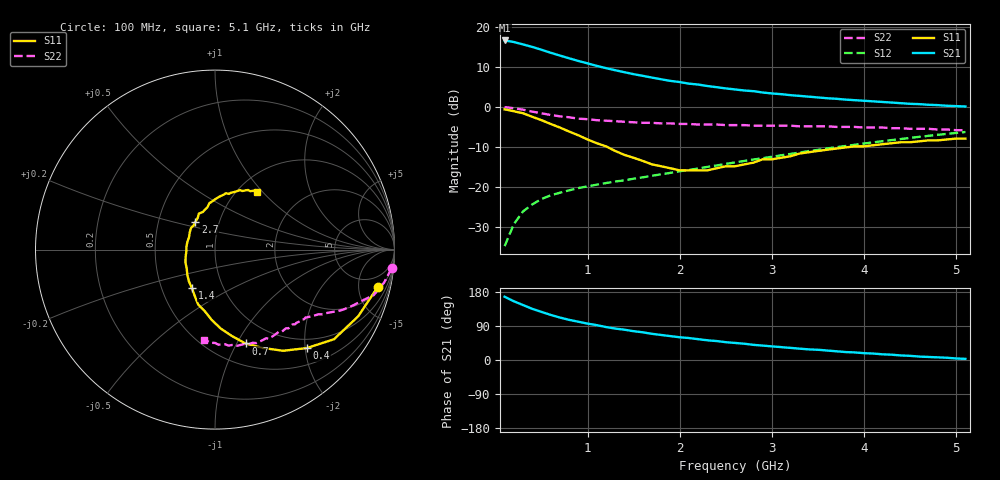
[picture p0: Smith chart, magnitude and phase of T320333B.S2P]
!AT-32033
!S and NOISE PARAMETERS at Vce=2.7V  Ic=2mA.  LAST UPDATED 01-05-95
# ghz s ma r 50
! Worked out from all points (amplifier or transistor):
!   51 points, 100 MHz to 5.1 GHz, reference 50 ohm
!   highest |S21| = 16.6 dB at 100 MHz (marker M1)
!   |S21| within 3 dB of that: start of sweep to 589.7 MHz
!   unconditionally stable (mu >= 1): 1.71 GHz to 2.774 GHz
!   at 900 MHz: K = 0.72, MSG = 15.9 dB, |S12| = -20.4 dB
!   at 2.6 GHz: K = 1.02, MAG = 8.3 dB, |S12| = -13.9 dB
!   at 5.1 GHz: K = 0.86, MSG = 3.2 dB, |S12| = -6.3 dB
!   lowest NFmin = 0.57 dB at 500 MHz
!   S11 on the Smith chart (normalised r, x): 100 MHz: 2.57, -7.96; 400 MHz: 0.81, -2.03; 700 MHz: 0.72, -1.09; 1.4 GHz: 0.71, -0.32; 2.7 GHz: 0.77, +0.25; 5.1 GHz: 1.22, +0.94
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0.1  0.93 -13.0  6.77 167.0  0.018 82.0  0.99 -6.0
0.2  0.88 -25.0  6.47 155.0  0.034 75.0  0.96 -11.0
0.3  0.83 -37.0  6.04 145.0  0.049 69.0  0.92 -16.0
0.4  0.75 -47.0  5.62 135.0  0.06 65.0  0.87 -19.0
0.5  0.68 -56.0  5.18 127.0  0.07 61.0  0.83 -22.0
0.6  0.61 -64.0  4.75 119.0  0.078 59.0  0.79 -25.0
0.7  0.55 -72.0  4.38 112.0  0.084 57.0  0.76 -27.0
0.8  0.49 -79.0  4.05 106.0  0.09 55.0  0.74 -28.0
1  0.39 -93.0  3.5 96.0  0.101 54.0  0.7 -31.0
1.2  0.32 -107.0  3.05 87.0  0.111 54.0  0.67 -33.0
1.3  0.28 -114.0  2.87 83.0  0.116 54.0  0.66 -34.0
1.4  0.25 -121.0  2.71 80.0  0.12 55.0  0.65 -35.0
1.5  0.23 -129.0  2.56 76.0  0.126 55.0  0.64 -36.0
1.8  0.18 -156.0  2.21 66.0  0.143 57.0  0.62 -39.0
2.2  0.16 164.0  1.9 55.0  0.169 58.0  0.6 -44.0
2.6  0.18 131.0  1.65 45.0  0.201 58.0  0.59 -49.0
2.7  0.19 125.0  1.6 43.0  0.21 58.0  0.59 -51.0
3  0.22 108.0  1.47 36.0  0.237 57.0  0.58 -56.0
3.5  0.28 90.0  1.31 27.0  0.289 55.0  0.57 -64.0
3.8  0.31 81.0  1.23 21.0  0.323 53.0  0.56 -69.0
4.3  0.35 69.0  1.13 14.0  0.383 48.0  0.54 -79.0
5.1  0.4 54.0  1.01 3.0  0.484 38.0  0.51 -97.0
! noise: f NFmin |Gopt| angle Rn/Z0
0.5  0.57  0.77  15  0.36
0.9  0.78  0.63  49  0.28
1.8  1.25  0.32  136  0.1
2.4  1.57  0.4  -159  0.08
